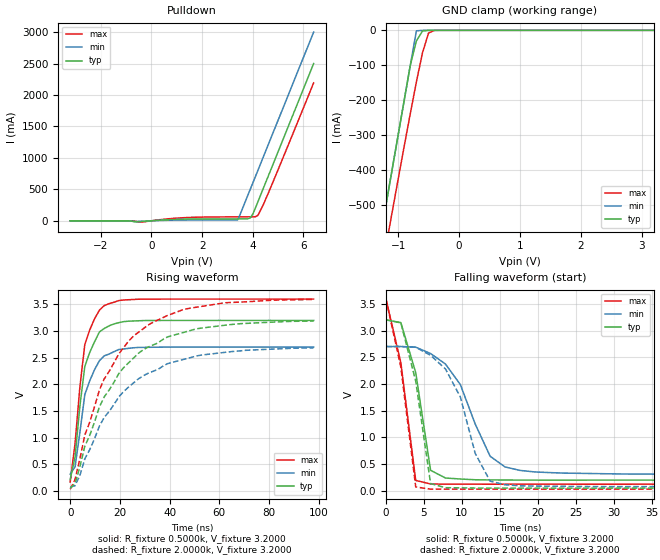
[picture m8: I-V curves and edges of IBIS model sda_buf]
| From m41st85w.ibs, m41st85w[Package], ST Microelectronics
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|   Model sda_buf
[Model]   sda_buf
Model_type   I/O_open_drain
Polarity   Non-Inverting
Enable   Active-High
Vinl =   0.3000V
Vinh =   0.7000V
Vmeas =   1.5000V
Cref =  50.0000pF
Rref =   0.3330k
Vref =   1.7500V
C_comp   12.0100pF   11.6900pF   12.2500pF
[Temperature Range]   27.0000   85.0000   -40.0000
[Voltage Range]   3.2000V   2.7000V   3.6000V
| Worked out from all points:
|   slope of the pulldown table from 0 to 0.48 V, typ, clamps not added: 36.6 ohm
|   GND clamp passes 1 mA (typ) near -0.55 V on its own axis
|   rising waveform, R_fixture 0.5000k, V_fixture 3.2000: 20-80 % time 5.59ns typ, 6.32ns min, 5.22ns max; typ from 0.22 V to 3.2 V
|   rising waveform, R_fixture 2.0000k, V_fixture 3.2000: 20-80 % time 21.9ns typ, 23.6ns min, 20.4ns max; typ from 0.052 V to 3.19 V
|   falling waveform, R_fixture 0.5000k, V_fixture 3.2000: 20-80 % time 2.33ns typ, 4.66ns min, 2.22ns max; typ from 3.2 V to 0.199 V
|   falling waveform, R_fixture 2.0000k, V_fixture 3.2000: 20-80 % time 2.33ns typ, 3.9ns min, 2.24ns max; typ from 3.2 V to 0.05 V
[Pulldown]
| voltage   I(typ)   I(min)   I(max)
-3.2V     0A         0A         -200uA
-800mV    -4.36mA    0A         -2.64mA
-400mV    -12.66mA   -7.235mA   -22.17mA
1.2V      24.99mA    11.75mA    47.43mA
3.4V      30.47mA    13.72mA    62.33mA
3.8V      31.28mA    400mA      62.81mA
3.9V      46.06mA    500mA      62.93mA
4V        105.2mA    600mA      63.05mA
4.2V      300mA      800mA      84.98mA
4.4V      500mA      1A         242.6mA
4.8V      900mA      1.4A       619.9mA
6.4V      2.5A       3A         2.193A
[GND_clamp]
| voltage   I(typ)   I(min)   I(max)
-3.2V     -2.5A      -2.5A      -2.59A
-1.3V     -600mA     -600mA     -716mA
-1.2V     -500mA     -500mA     -619mA
-1.1V     -400mA     -400mA     -522.4mA
-800mV    -100mA     -100mA     -238.3mA
-700mV    -30.38mA   -1.4mA     -147.9mA
-600mV    -2.04mA    -108.9uA   -64.5mA
-500mV    -68.31uA   -14.93uA   -7.62mA
-400mV    -3.222uA   -2.477uA   -79.64uA
3.2V      86.03pA    1.819uA    78.36pA
[Ramp]
| variable   typ   min   max
dV/dt_r   1.7403/3.8302n   1.3401/4.2065n   2.0486/3.5272n
dV/dt_f   1.7403/2.1489n   1.3401/5.4133n   2.0487/1.1044n
R_load = 0.3330k
[Rising Waveform]
R_fixture = 0.5000k
V_fixture = 3.2000
V_fixture_min = 2.7000
V_fixture_max = 3.6000
| time   V(typ)   V(min)   V(max)
0s        219.9mV    319.7mV    172.9mV
1.96ns    639.9mV    457.2mV    893.9mV
3.92ns    1.601V     1.107V     1.963V
5.88ns    2.338V     1.81V      2.748V
9.8ns     2.8V       2.277V     3.23V
11.76ns   2.984V     2.444V     3.393V
13.72ns   3.049V     2.537V     3.478V
19.6ns    3.158V     2.655V     3.573V
27.44ns   3.193V     2.693V     3.597V
98ns      3.2V       2.7V       3.6V
[Rising Waveform]
R_fixture = 2.0000k
V_fixture = 3.2000
V_fixture_min = 2.7000
V_fixture_max = 3.6000
| time   V(typ)   V(min)   V(max)
0s        51.83mV    77.95mV    37.46mV
1.96ns    142.3mV    102.5mV    221.4mV
5.88ns    842mV      604.9mV    1.053V
11.76ns   1.579V     1.22V      1.895V
19.6ns    2.206V     1.769V     2.575V
25.48ns   2.494V     2.028V     2.906V
39.2ns    2.891V     2.39V      3.293V
47.04ns   2.994V     2.486V     3.42V
66.64ns   3.131V     2.622V     3.54V
98ns      3.189V     2.686V     3.592V
[Falling Waveform]
R_fixture = 0.5000k
V_fixture = 3.2000
V_fixture_min = 2.7000
V_fixture_max = 3.6000
| time   V(typ)   V(min)   V(max)
0s        3.2V       2.7V       3.589V
1.96ns    3.148V     2.7V       2.399V
3.92ns    2.212V     2.688V     193.8mV
5.88ns    383.5mV    2.569V     127.3mV
7.84ns    239.2mV    2.372V     124.2mV
9.8ns     220.5mV    1.988V     123.8mV
11.76ns   206.5mV    1.249V     123.5mV
13.72ns   203.3mV    647.3mV    123.4mV
17.64ns   200.7mV    381.9mV    123.5mV
98ns      199.2mV    309.9mV    123.5mV
[Falling Waveform]
R_fixture = 2.0000k
V_fixture = 3.2000
V_fixture_min = 2.7000
V_fixture_max = 3.6000
| time   V(typ)   V(min)   V(max)
0s        3.2V       2.7V       3.589V
1.96ns    3.143V     2.7V       2.311V
3.92ns    2.052V     2.686V     71.99mV
5.88ns    134.3mV    2.536V     31.35mV
7.84ns    57.74mV    2.28V      31.48mV
9.8ns     55.49mV    1.756V     30.98mV
11.76ns   51.29mV    698.7mV    30.33mV
13.72ns   50.47mV    181.2mV    30.78mV
15.68ns   50.56mV    112.3mV    31.11mV
98ns      49.63mV    76.59mV    31.15mV
